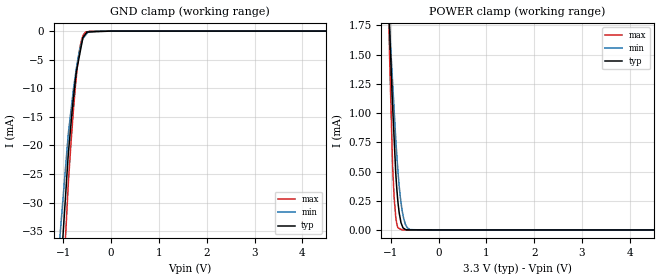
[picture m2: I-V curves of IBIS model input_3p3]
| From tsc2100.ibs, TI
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|   input_3p3 Model
[Model]   input_3p3
Model_type   Input
Vinl = 0.99
Vinh = 2.31
|   typ   min   max
|   (nom PVT)   (fast PVT)   (slow PVT)
|C_comp from frequency sweep method (F=50MHz)
|Average
|C_comp   1.239e-12   1.232e-12   1.241e-12
|C_comp from LC tank measurement(L=1nH)
|Average
|Resonant Frequency(Hz)   5.090e+09   5.110e+09   5.089e+09
C_comp   9.787e-13   9.710e-13   9.790e-13
| Where nom  PVT is Nominal Process, 3.3V, 26C
|   Fast PVT is Strong Process,  3.6V, -40C
|   Slow PVT is Weak Process,   3V, 86C
[Model Spec]
|Subparameter   typ   min   max
Vinh   2.31   2.1   2.52
Vinl   0.99   0.9   1.08
[Voltage Range]   3.3   3   3.6
|Ambient Temperature   25   85   -40
|Junction Temperature
[Temperature Range]   26   86   -40
[Power Clamp Reference]   3.3   3   3.6
[GND Clamp Reference]   0   0   0
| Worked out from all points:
|   GND clamp passes 1 mA (typ) near -0.58 V on its own axis
|   POWER clamp passes 1 mA (typ) near -0.96 V on its own axis
[GND Clamp]
|   Voltage   I(typ)   I(min)   I(max)
-3.3V     -1.787A    -1.624A    -1.965A
-1.498V   -98.84mA   -79.64mA   -123.5mA
-897.6mV  -21.51mA   -18.01mA   -26.74mA
-792mV    -11.87mA   -10.32mA   -14.02mA
-726mV    -6.993mA   -6.382mA   -7.792mA
-702mV    -5.949mA   -5.157mA   -5.815mA
-658.8mV  -4.069mA   -3.33mA    -3.124mA
-622.8mV  -2.503mA   -2.127mA   -1.616mA
-590.7mV  -1.106mA   -1.296mA   -839.1uA
-532.8mV  -471.1uA   -685.4uA   -172.5uA
-285mV    -92.69uA   -1.053uA   -3.877uA
6.6V      0A         0A         0A
[POWER Clamp]
|   Voltage   I(typ)   I(min)   I(max)
-3.3V     32.16mA    22.45mA    56.05mA
-1.073V   2.254mA    2.104mA    2.407mA
-1.03V    1.754mA    1.751mA    1.532mA
-1.026V   1.715mA    1.722mA    1.468mA
-964.8mV  1.065mA    1.269mA    561.5uA
-932.4mV  784.7uA    1.029mA    280.4uA
-897.6mV  483.4uA    771uA      109.9uA
-861.3mV  278.2uA    551.5uA    29.15uA
-766.8mV  39.59uA    171.4uA    409.3nA
-696mV    4.262uA    47.76uA    320.9nA
-591mV    797.3nA    2.894uA    189.7nA
6.6V      0A         0A         0A
